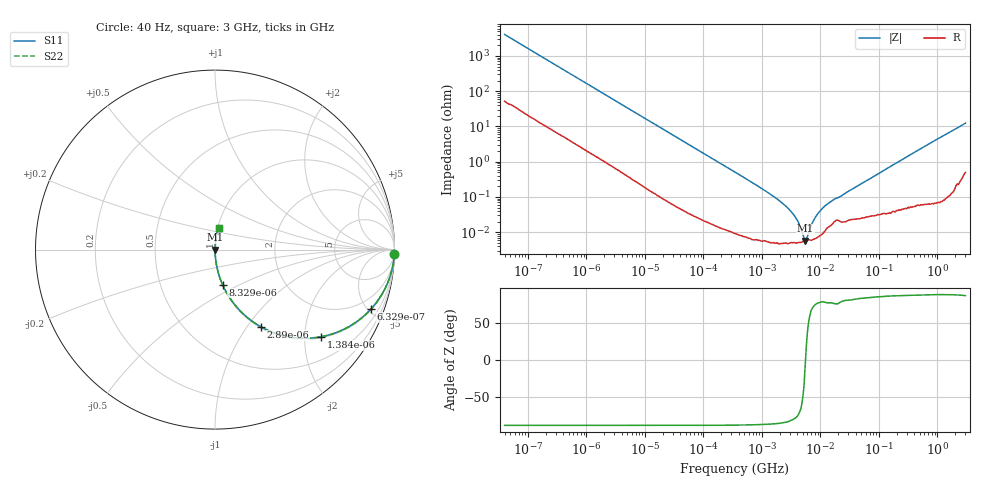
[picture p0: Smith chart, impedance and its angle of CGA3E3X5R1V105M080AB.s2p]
! S-parameter Generated by TDK Corporation
! Copyright(C) 2015 TDK Corporation.
! All Rights Reserved.
! TDK P/N: CGA3E3X5R1V105M080AB (Multilayer Ceramic Chip Capacitors)
! Property: C=1uF
! Size(LxWxT): 1.6x0.8x0.8mm, 0.063x0.031x0.031inches
! Model Type: s2p (Touchstone File Format Version 1.0)
! Frequency: DC=Yes Start=0.00004MHz Stop=3000MHz 396points Log-sweep
! Note: This model was converted from impedance.
! Model Generated on Jun. 23, 2015
! Hash(MD5):
! Port Assignments:
!  1 ---| |--- 2
! Applicable Conditions:
!  Temperature = 25 degC
!  DC Bias Voltage = 0 V
!  Small Signal Operation
! Terms and conditions regarding TDK Simulation Models
! (1)This simulation model is being provided solely for informational purposes. Please refer to the specifications of the products in terms of detailed characteristics of such products.
! (2)In no event shall TDK Corporation of any of its subsidiaries be liable for any loss or damage arising, directly or indirectly,
!  From any information contained in this simulation model, including, but not limited to loss or damages arising from any inaccuracies, omissions or errors in connection with such information.
! (3)Any and all copyrights on this simulation model are owned by TDK Corporation.
!  Duplication or redistribution of this simulation model without prior written permission from TDK Corporation is prohibited.
! (4)This simulation model is subject to any modification or change without any prior notice.
! (5)Neither TDK Corporation nor any of its subsidiaries shall make any warranty, express or implied,
!  Including but not limited to the correctness, implied warranties of merchantability and fitness for a particular purpose with respect to this simulation models.
! (6)The use of this simulation model shall be deemed to have consented to the terms and conditions hereof.
# MHz S MA R 50
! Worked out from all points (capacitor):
!   395 points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, 40 Hz to 3 GHz, reference 50 ohm
!   read as one part in series: C = 978 nF near 41.88 Hz
!   lowest |Z| = 5.72 mohm at 5.481 MHz (marker M1)
!   series resonance near 5.561 MHz, so ESL is about 840 pH
!   S11 on the Smith chart (normalised r, x): 40 Hz: 2, -81; 632.9 Hz: 1.06, -5.24; 1.384 kHz: 1.03, -2.41; 2.89 kHz: 1.01, -1.16; 8.329 kHz: 1.00, -0.41; 3 GHz: 1.01, +0.25
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4e-05  0.9994 -1.4  0.02456 87.9  0.02456 87.9  0.9994 -1.4
0.0001912643  0.9919 -6.6  0.1154 82.7  0.1154 82.7  0.9919 -6.6
0.0006328604  0.9304 -20.8  0.3553 68.5  0.3553 68.5  0.9304 -20.8
0.000834128  0.8892 -26.5  0.4468 62.8  0.4468 62.8  0.8892 -26.5
0.001383868  0.7648 -39.4  0.6349 49.9  0.6349 49.9  0.7648 -39.4
0.002889976  0.4993 -59.4  0.8604 30.0  0.8604 30.0  0.4993 -59.4
0.004578982  0.344 -69.2  0.935 20.1  0.935 20.1  0.344 -69.2
0.008329251  0.1992 -77.9  0.9778 11.5  0.9778 11.5  0.1992 -77.9
0.01739424  0.0979 -83.8  0.9942 5.6  0.9942 5.6  0.0979 -83.8
0.3464102  0.005057 -88.7  0.9999 0.3  0.9999 0.3  0.005057 -88.7
1.200196  0.001411 -87.7  0.9999 0.1  0.9999 0.1  0.001411 -87.7
2.286002  0.0006473 -85.7  1 0.0  1 0.0  0.0006473 -85.7
3.792615  0.0002561 -78.9  1 0.0  1 0.0  0.0002561 -78.9
4.773931  0.0001099 -61.6  0.9999 0.0  0.9999 0.0  0.0001099 -61.6
5.480732  5.716e-05 -8.9  0.9999 0.0  0.9999 0.0  5.716e-05 -8.9
6.292177  9.835e-05 52.3  0.9999 -0.0  0.9999 -0.0  9.835e-05 52.3
7.22376  0.0001789 70.5  0.9999 -0.0  0.9999 -0.0  0.0001789 70.5
9.521122  0.000374 78.1  0.9999 -0.0  0.9999 -0.0  0.000374 78.1
13.75903  0.0006646 77.8  0.9999 -0.0  0.9999 -0.0  0.0006646 77.8
150.6385  0.007023 86.7  0.9996 -0.4  0.9996 -0.4  0.007023 86.7
906.6656  0.04001 86.8  0.9985 -2.3  0.9985 -2.3  0.04001 86.8
3000  0.1221 80.7  0.9876 -7.0  0.9876 -7.0  0.1221 80.7
